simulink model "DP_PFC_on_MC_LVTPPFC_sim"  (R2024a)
settings: Solver=odeN  StartTime=0.0  StopTime=1  FixedStep=Ts  MaxStep=10e-6  RelTol=1e-3  AbsTol=1e-4  EnableMultiTasking=on
PreLoadFcn:
  | TotemPole_PFCData;
StopFcn:
  | out.getSimulationMetadata.TimingInfo
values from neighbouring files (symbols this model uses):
  PWM = PWMType.Implementation    [TotemPole_PFCData.m]
  Ts = 5e-9    (= 5e-09)    [TotemPole_PFCData.m]
  Tsc_fast = 1e-5    (= 1e-05)    [TotemPole_PFCData.m]
  Tsc_slow = 0.01    [TotemPole_PFCData.m]
  Vrms = 23.0    (= 23)    [TotemPole_PFCData.m]
undefined symbols (not defined in the file or in its folder): AC, ADCs, ClosedLoop, Const, Detailed, Implementation, Inversion, Microchip, Noise, PI, Rnom, Simulation, ZenerResistiveLoad
libraries: fl_lib x23, nesl_utility x15, ee_lib x11, simulink x8, slctrl_fre x1, eeTotalHarmonicDistorsion x1
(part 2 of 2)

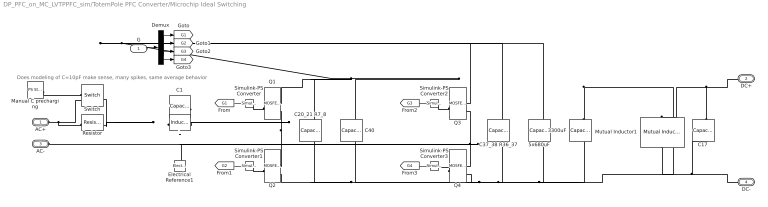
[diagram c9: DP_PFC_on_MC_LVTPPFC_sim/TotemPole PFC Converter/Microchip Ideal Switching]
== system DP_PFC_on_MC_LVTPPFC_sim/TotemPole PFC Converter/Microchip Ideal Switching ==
  note: Does modeling of C=10pF make sense, many spikes, same average behavior
  G : Inport
  3300uF : fl_lib/Electrical/Electrical Elements/Capacitor  c=3300 uF  r=65 mOhm  g=0 1/Ohm  i_specify=off  i_priority=None  i=0 A  i_nominal_specify=off  i_nominal_value=1  i_nominal_unit=A  v_specify=off  v_priority=High  v=0.1 V  v_nominal_specify=off  v_nominal_value=1  v_nominal_unit=V  vc_specify=off  vc_priority=High  vc=0 V  vc_nominal_specify=off  vc_nominal_value=1  vc_nominal_unit=V
  5x680uF : fl_lib/Electrical/Electrical Elements/Capacitor  c=680*5 uF  r=90/5 mOhm  g=0 1/Ohm  i_specify=off  i_priority=None  i=0 A  i_nominal_specify=off  i_nominal_value=1  i_nominal_unit=A  v_specify=off  v_priority=High  v=0.1 V  v_nominal_specify=off  v_nominal_value=1  v_nominal_unit=V  vc_specify=off  vc_priority=High  vc=0 V  vc_nominal_specify=off  vc_nominal_value=1  vc_nominal_unit=V
  C1 : fl_lib/Electrical/Electrical Elements/Capacitor  Commented=on  c=10 pF  r=0 Ohm  g=0 1/Ohm  i_specify=off  i_priority=None  i=0 A  i_nominal_specify=off  i_nominal_value=1  i_nominal_unit=A  v_specify=off  v_priority=High  v=0.1 V  v_nominal_specify=off  v_nominal_value=1  v_nominal_unit=V  vc_specify=off  vc_priority=High  vc=0 V  vc_nominal_specify=off  vc_nominal_value=1  vc_nominal_unit=V
  C17 : fl_lib/Electrical/Electrical Elements/Capacitor  c=2 uF  r=0 mOhm  g=0 1/Ohm  i_specify=off  i_priority=None  i=0 A  i_nominal_specify=off  i_nominal_value=1  i_nominal_unit=A  v_specify=off  v_priority=High  v=0.1 V  v_nominal_specify=off  v_nominal_value=1  v_nominal_unit=V  vc_specify=off  vc_priority=High  vc=0 V  vc_nominal_specify=off  vc_nominal_value=1  vc_nominal_unit=V
  C20_21 R7_8 : fl_lib/Electrical/Electrical Elements/Capacitor  c=44 nF  r=7.5 Ohm  g=0 1/Ohm  i_specify=off  i_priority=None  i=0 A  i_nominal_specify=off  i_nominal_value=1  i_nominal_unit=A  v_specify=off  v_priority=High  v=0.1 V  v_nominal_specify=off  v_nominal_value=1  v_nominal_unit=V  vc_specify=off  vc_priority=High  vc=0 V  vc_nominal_specify=off  vc_nominal_value=1  vc_nominal_unit=V
  C37_38 R36_37 : fl_lib/Electrical/Electrical Elements/Capacitor  c=44 nF  r=7.5 Ohm  g=0 1/Ohm  i_specify=off  i_priority=None  i=0 A  i_nominal_specify=off  i_nominal_value=1  i_nominal_unit=A  v_specify=off  v_priority=High  v=0.1 V  v_nominal_specify=off  v_nominal_value=1  v_nominal_unit=V  vc_specify=off  vc_priority=High  vc=0 V  vc_nominal_specify=off  vc_nominal_value=1  vc_nominal_unit=V
  C40 : fl_lib/Electrical/Electrical Elements/Capacitor  c=2 uF  r=0 mOhm  g=0 1/Ohm  i_specify=off  i_priority=None  i=0 A  i_nominal_specify=off  i_nominal_value=1  i_nominal_unit=A  v_specify=off  v_priority=High  v=0.1 V  v_nominal_specify=off  v_nominal_value=1  v_nominal_unit=V  vc_specify=off  vc_priority=High  vc=0 V  vc_nominal_specify=off  vc_nominal_value=1  vc_nominal_unit=V
  Demux : Demux
  Electrical Reference1 : fl_lib/Electrical/Electrical Elements/Electrical Reference
  L : fl_lib/Electrical/Electrical Elements/Inductor  l=266 uH  r=18 mOhm  g=0 1/Ohm  i_specify=off  i_priority=None  i=0 A  i_nominal_specify=off  i_nominal_value=1  i_nominal_unit=A  v_specify=off  v_priority=None  v=0 V  v_nominal_specify=off  v_nominal_value=1  v_nominal_unit=V  i_L_specify=off  i_L_priority=High  i_L=0 A  i_L_nominal_specify=off  i_L_nominal_value=1  i_L_nominal_unit=A
  Manual C precharging : fl_lib/Physical Signals/Sources/PS Step  step_time=0.10 ms  initial_value=1  final_value=0
  Mutual Inductor1 : ee_lib/Passive/Transformers/Mutual Inductor  L1=4.7 uH  L2=4.7 uH  k=0.9  L_tol=0  enable_L1_tol=ee.enum.toleranceApplication.none  L1_tol_distribution=ee.enum.toleranceDistribution.uniform  L1_nSigma=4  enable_L2_tol=ee.enum.toleranceApplication.none  L2_tol_distribution=ee.enum.toleranceDistribution.uniform  L2_nSigma=4  r=[4,4] mOhm  g=[1e-8,1e-8] 1/Ohm  enable_operating_limits=ee.enum.enable.no  operating_limit_action=ee.enum.passive.reportOpLim.warn  max_working_current=1 A  power_rating=1 W  enable_faults=ee.enum.enable.no  fault_action=simscape.enum.assert.action.none  fault_winding=ee.enum.passive.transformers.faultedWinding.primary  lambdaPercent=50  turnsShort=ee.enum.faults.faultTurnsShort.no  openCct=ee.enum.faults.faultTurnsOpenCkt.no  groundShort=ee.enum.faults.faultTurnsGroundShort.no  groundShortG=0 1/Ohm  tau_fault=1e-3 s  fault_trigger=ee.enum.faults.faultTrigger.temporal  t_fault=1 s  max_permissible_voltage=100 V  n_fail_on_voltage=1  max_permissible_current=1 A  t_fail_on_current=1 s  iL1_specify=off  iL1_priority=High  iL1=0 A  iL1_nominal_specify=off  iL1_nominal_value=1  iL1_nominal_unit=A  iL2_specify=off  iL2_priority=High  iL2=0 A  iL2_nominal_specify=off  iL2_nominal_value=1  iL2_nominal_unit=A  faulted_specify=off  faulted_priority=None  faulted=0
  Q1 : ee_lib/Semiconductors & Converters/MOSFET (Ideal, Switching)  port_option=ee.enum.controlport.ps  Rds=0.034 Ohm  Goff=1e-5 1/Ohm  Vth=0.5 V  diode_param=2  diode_Vf=3 V  diode_Ron=0.3 Ohm  diode_Goff=4e-5 1/Ohm  diode_C=50e-9 F  diode_iRM=-235 A  diode_iF=300 A  diode_idot=-50 A/us  diode_trr_param=1  diode_trr_factor=3  diode_trr=15 us  diode_Qrr=1500 s*uA  ids_specify=off  ids_priority=None  ids=0 A  ids_nominal_specify=off  ids_nominal_value=1  ids_nominal_unit=A  vds_specify=off  vds_priority=None  vds=0 V  vds_nominal_specify=off  vds_nominal_value=1  vds_nominal_unit=V  vgs_specify=off  vgs_priority=None  vgs=0 V  vgs_nominal_specify=off  vgs_nominal_value=1  vgs_nominal_unit=V  thermal_loss_option=ee.enum.converters.thermalLossOption.constantvalues  Von_data=[0, 1.8, 3.2, 6, 10, 16; 0, 2, 5.5, 9.5, 15, 25] V  Tj=[298.15, 448.15] K  Iout_data=[0, 20, 40, 60, 80, 100] A  Eon_data=[0, 55.04, 124.57, 235.53, 362.12; 0, 71.25, 161.25, 304.88, 468.75] * 1e-6 J  Eoff_data=[0, 18, 30, 56.1, 76.5; 0, 22.5, 37.5, 70.13, 95.63] * 1e-6 J  Eon_data_3D=[zeros(2, 5, 3)] J  Eoff_data_3D=[zeros(2, 5, 3)] J  Tj_loss=[298.15, 448.15] K  Iout_data_loss=[0, 10, 20, 30, 40] A  tabulateWithVds=false  Vds_loss=[0, 150, 300] V  Eon_scalar=22.86e-3 J  Eoff_scalar=17.14e-3 J  Voff=300 V  Iout_scalar=600 A  useCurrentFromPreviousCycle=false  useVoltageFromPreviousCycle=false  diodeModelType=ee.enum.converters.diodeModelType.pwl  diodeTableType=ee.enum.diode.tableType.IfMat  diode_ReverseIVType=ee.enum.diode.diodeReverseIV.constant  diode_IfMat=[.07, .12, .19, 1.75, 4.24, 7.32, 11.2; .16, .3, .72, 2.14, 4.02, 6.35, 9.12] A  diode_VfMat=[.9, 1.15, 1.25, 1.5, 1.75, 2.17, 2.6, 2.85; .58, .68, .75, 1.1, 1.38, 1.77, 2.27, 2.7] V  diode_TjVec=[25, 125] degC  diode_VfVec=[.5, .7, .9, 1.3, 1.7, 2.1, 2.5] V  diode_IfVec=[.1, .2, .5, 1, 2, 4, 7, 10] A  diode_IrMat=[1e-06, 2e-06, 5e-06, 1e-05, 2.5e-05, 5e-05, .0001; 2e-06, 5e-06, 1e-05, 4e-05, 8e-05, .0002, .0005] A  diode_VrMat=[10, 100, 200, 250, 300, 325, 350; 10, 70, 160, 220, 270, 300, 320] V  diode_VrVec=[10, 20, 40, 50, 70, 80, 100] V  diode_IrVec=[1e-06, 2e-06, 5e-06, 1e-05, 2e-05, 5e-05, .0001] A  diode_Vr=-600 V  diode_Ls=150 nH  diode_Erec=0.03 J  diode_rec_loss_model=ee.enum.diode.reverseRecoveryModel.fixed  diode_ErecVal=0 J  diode_scaleWithIandV=true  diode_ErecMat=zeros(2, 3) J  diode_TjrecVec=[298.15, 398.15] K  diode_IfrecVec=[.1, 1, 10] A  diode_IrecVal=10 A  diode_VrecVal=10 V  diode_tFilter=1 / 1000 / 100 s  thermal_network_parameterization=ee.enum.thermalNetworkTopology.external  Rth=[.03, .2] K/W  Rth_Cauer=[.03, .1, .2] K/W  Rth_Foster=[.03, .2] K/W  thermal_mass_parameterization=ee.enum.thermalNetwork.timeconstant  thermal_mass=[3, 25] J/K  thermal_mass_Cauer=[3, 10, 25] J/K  thermal_mass_Foster=[33, 50] J/K  thermal_time_constant=[.1, 5] s  thermal_time_constant_Cauer=[.1, 1, 5] s  thermal_time_constant_Foster=[1, 10] s  thermal_mass_initial_temperatures=[25, 25] degC  thermal_mass_initial_temperatures_Cauer=[25, 25, 25] degC  junction_thermal_mass=0.1 J/K  Tvec_initial_Foster=[25, 25, 25, 25] degC  no_thermal_network=0  junction_temperature_specify=off  junction_temperature_priority=None  junction_temperature=25 degC  junction_temperature_nominal_specify=off  junction_temperature_nominal_value=1  junction_temperature_nominal_unit=degC  Qj_specify=off  Qj_priority=None  Qj=0 W  Qj_nominal_specify=off  Qj_nominal_value=1  Qj_nominal_unit=W  accumulatedSwitchingLosses_specify=off  accumulatedSwitchingLosses_priority=None  accumulatedSwitchingLosses=0 J
  Q2 : ee_lib/Semiconductors & Converters/MOSFET (Ideal, Switching)  port_option=ee.enum.controlport.ps  Rds=0.034 Ohm  Goff=1e-5 1/Ohm  Vth=0.5 V  diode_param=2  diode_Vf=3 V  diode_Ron=0.3 Ohm  diode_Goff=4e-5 1/Ohm  diode_C=50e-9 F  diode_iRM=-235 A  diode_iF=300 A  diode_idot=-50 A/us  diode_trr_param=1  diode_trr_factor=3  diode_trr=15 us  diode_Qrr=1500 s*uA  ids_specify=off  ids_priority=None  ids=0 A  ids_nominal_specify=off  ids_nominal_value=1  ids_nominal_unit=A  vds_specify=off  vds_priority=None  vds=0 V  vds_nominal_specify=off  vds_nominal_value=1  vds_nominal_unit=V  vgs_specify=off  vgs_priority=None  vgs=0 V  vgs_nominal_specify=off  vgs_nominal_value=1  vgs_nominal_unit=V  thermal_loss_option=ee.enum.converters.thermalLossOption.constantvalues  Von_data=[0, 1.8, 3.2, 6, 10, 16; 0, 2, 5.5, 9.5, 15, 25] V  Tj=[298.15, 448.15] K  Iout_data=[0, 20, 40, 60, 80, 100] A  Eon_data=[0, 55.04, 124.57, 235.53, 362.12; 0, 71.25, 161.25, 304.88, 468.75] * 1e-6 J  Eoff_data=[0, 18, 30, 56.1, 76.5; 0, 22.5, 37.5, 70.13, 95.63] * 1e-6 J  Eon_data_3D=[zeros(2, 5, 3)] J  Eoff_data_3D=[zeros(2, 5, 3)] J  Tj_loss=[298.15, 448.15] K  Iout_data_loss=[0, 10, 20, 30, 40] A  tabulateWithVds=false  Vds_loss=[0, 150, 300] V  Eon_scalar=22.86e-3 J  Eoff_scalar=17.14e-3 J  Voff=300 V  Iout_scalar=600 A  useCurrentFromPreviousCycle=false  useVoltageFromPreviousCycle=false  diodeModelType=ee.enum.converters.diodeModelType.pwl  diodeTableType=ee.enum.diode.tableType.IfMat  diode_ReverseIVType=ee.enum.diode.diodeReverseIV.constant  diode_IfMat=[.07, .12, .19, 1.75, 4.24, 7.32, 11.2; .16, .3, .72, 2.14, 4.02, 6.35, 9.12] A  diode_VfMat=[.9, 1.15, 1.25, 1.5, 1.75, 2.17, 2.6, 2.85; .58, .68, .75, 1.1, 1.38, 1.77, 2.27, 2.7] V  diode_TjVec=[25, 125] degC  diode_VfVec=[.5, .7, .9, 1.3, 1.7, 2.1, 2.5] V  diode_IfVec=[.1, .2, .5, 1, 2, 4, 7, 10] A  diode_IrMat=[1e-06, 2e-06, 5e-06, 1e-05, 2.5e-05, 5e-05, .0001; 2e-06, 5e-06, 1e-05, 4e-05, 8e-05, .0002, .0005] A  diode_VrMat=[10, 100, 200, 250, 300, 325, 350; 10, 70, 160, 220, 270, 300, 320] V  diode_VrVec=[10, 20, 40, 50, 70, 80, 100] V  diode_IrVec=[1e-06, 2e-06, 5e-06, 1e-05, 2e-05, 5e-05, .0001] A  diode_Vr=-600 V  diode_Ls=150 nH  diode_Erec=0.03 J  diode_rec_loss_model=ee.enum.diode.reverseRecoveryModel.fixed  diode_ErecVal=0 J  diode_scaleWithIandV=true  diode_ErecMat=zeros(2, 3) J  diode_TjrecVec=[298.15, 398.15] K  diode_IfrecVec=[.1, 1, 10] A  diode_IrecVal=10 A  diode_VrecVal=10 V  diode_tFilter=1 / 1000 / 100 s  thermal_network_parameterization=ee.enum.thermalNetworkTopology.external  Rth=[.03, .2] K/W  Rth_Cauer=[.03, .1, .2] K/W  Rth_Foster=[.03, .2] K/W  thermal_mass_parameterization=ee.enum.thermalNetwork.timeconstant  thermal_mass=[3, 25] J/K  thermal_mass_Cauer=[3, 10, 25] J/K  thermal_mass_Foster=[33, 50] J/K  thermal_time_constant=[.1, 5] s  thermal_time_constant_Cauer=[.1, 1, 5] s  thermal_time_constant_Foster=[1, 10] s  thermal_mass_initial_temperatures=[25, 25] degC  thermal_mass_initial_temperatures_Cauer=[25, 25, 25] degC  junction_thermal_mass=0.1 J/K  Tvec_initial_Foster=[25, 25, 25, 25] degC  no_thermal_network=0  junction_temperature_specify=off  junction_temperature_priority=None  junction_temperature=25 degC  junction_temperature_nominal_specify=off  junction_temperature_nominal_value=1  junction_temperature_nominal_unit=degC  Qj_specify=off  Qj_priority=None  Qj=0 W  Qj_nominal_specify=off  Qj_nominal_value=1  Qj_nominal_unit=W  accumulatedSwitchingLosses_specify=off  accumulatedSwitchingLosses_priority=None  accumulatedSwitchingLosses=0 J
  Q3 : ee_lib/Semiconductors & Converters/MOSFET (Ideal, Switching)  port_option=ee.enum.controlport.ps  Rds=0.24 Ohm  Goff=1e-5 1/Ohm  Vth=0.5 V  diode_param=2  diode_Vf=3.6 V  diode_Ron=0.066 Ohm  diode_Goff=4e-5 1/Ohm  diode_C=50e-9 F  diode_iRM=-235 A  diode_iF=300 A  diode_idot=-50 A/us  diode_trr_param=1  diode_trr_factor=3  diode_trr=15 us  diode_Qrr=1500 s*uA  ids_specify=off  ids_priority=None  ids=0 A  ids_nominal_specify=off  ids_nominal_value=1  ids_nominal_unit=A  vds_specify=off  vds_priority=None  vds=0 V  vds_nominal_specify=off  vds_nominal_value=1  vds_nominal_unit=V  vgs_specify=off  vgs_priority=None  vgs=0 V  vgs_nominal_specify=off  vgs_nominal_value=1  vgs_nominal_unit=V  thermal_loss_option=ee.enum.converters.thermalLossOption.constantvalues  Von_data=[0, 1.8, 3.2, 6, 10, 16; 0, 2, 5.5, 9.5, 15, 25] V  Tj=[298.15, 448.15] K  Iout_data=[0, 20, 40, 60, 80, 100] A  Eon_data=[0, 55.04, 124.57, 235.53, 362.12; 0, 71.25, 161.25, 304.88, 468.75] * 1e-6 J  Eoff_data=[0, 18, 30, 56.1, 76.5; 0, 22.5, 37.5, 70.13, 95.63] * 1e-6 J  Eon_data_3D=[zeros(2, 5, 3)] J  Eoff_data_3D=[zeros(2, 5, 3)] J  Tj_loss=[298.15, 448.15] K  Iout_data_loss=[0, 10, 20, 30, 40] A  tabulateWithVds=false  Vds_loss=[0, 150, 300] V  Eon_scalar=22.86e-3 J  Eoff_scalar=17.14e-3 J  Voff=300 V  Iout_scalar=600 A  useCurrentFromPreviousCycle=false  useVoltageFromPreviousCycle=false  diodeModelType=ee.enum.converters.diodeModelType.pwl  diodeTableType=ee.enum.diode.tableType.IfMat  diode_ReverseIVType=ee.enum.diode.diodeReverseIV.constant  diode_IfMat=[.07, .12, .19, 1.75, 4.24, 7.32, 11.2; .16, .3, .72, 2.14, 4.02, 6.35, 9.12] A  diode_VfMat=[.9, 1.15, 1.25, 1.5, 1.75, 2.17, 2.6, 2.85; .58, .68, .75, 1.1, 1.38, 1.77, 2.27, 2.7] V  diode_TjVec=[25, 125] degC  diode_VfVec=[.5, .7, .9, 1.3, 1.7, 2.1, 2.5] V  diode_IfVec=[.1, .2, .5, 1, 2, 4, 7, 10] A  diode_IrMat=[1e-06, 2e-06, 5e-06, 1e-05, 2.5e-05, 5e-05, .0001; 2e-06, 5e-06, 1e-05, 4e-05, 8e-05, .0002, .0005] A  diode_VrMat=[10, 100, 200, 250, 300, 325, 350; 10, 70, 160, 220, 270, 300, 320] V  diode_VrVec=[10, 20, 40, 50, 70, 80, 100] V  diode_IrVec=[1e-06, 2e-06, 5e-06, 1e-05, 2e-05, 5e-05, .0001] A  diode_Vr=-600 V  diode_Ls=150 nH  diode_Erec=0.03 J  diode_rec_loss_model=ee.enum.diode.reverseRecoveryModel.fixed  diode_ErecVal=0 J  diode_scaleWithIandV=true  diode_ErecMat=zeros(2, 3) J  diode_TjrecVec=[298.15, 398.15] K  diode_IfrecVec=[.1, 1, 10] A  diode_IrecVal=10 A  diode_VrecVal=10 V  diode_tFilter=1 / 1000 / 100 s  thermal_network_parameterization=ee.enum.thermalNetworkTopology.external  Rth=[.03, .2] K/W  Rth_Cauer=[.03, .1, .2] K/W  Rth_Foster=[.03, .2] K/W  thermal_mass_parameterization=ee.enum.thermalNetwork.timeconstant  thermal_mass=[3, 25] J/K  thermal_mass_Cauer=[3, 10, 25] J/K  thermal_mass_Foster=[33, 50] J/K  thermal_time_constant=[.1, 5] s  thermal_time_constant_Cauer=[.1, 1, 5] s  thermal_time_constant_Foster=[1, 10] s  thermal_mass_initial_temperatures=[25, 25] degC  thermal_mass_initial_temperatures_Cauer=[25, 25, 25] degC  junction_thermal_mass=0.1 J/K  Tvec_initial_Foster=[25, 25, 25, 25] degC  no_thermal_network=0  junction_temperature_specify=off  junction_temperature_priority=None  junction_temperature=25 degC  junction_temperature_nominal_specify=off  junction_temperature_nominal_value=1  junction_temperature_nominal_unit=degC  Qj_specify=off  Qj_priority=None  Qj=0 W  Qj_nominal_specify=off  Qj_nominal_value=1  Qj_nominal_unit=W  accumulatedSwitchingLosses_specify=off  accumulatedSwitchingLosses_priority=None  accumulatedSwitchingLosses=0 J
  Q4 : ee_lib/Semiconductors & Converters/MOSFET (Ideal, Switching)  port_option=ee.enum.controlport.ps  Rds=0.24 Ohm  Goff=1e-5 1/Ohm  Vth=0.5 V  diode_param=2  diode_Vf=3.6 V  diode_Ron=0.066 Ohm  diode_Goff=4e-5 1/Ohm  diode_C=50e-9 F  diode_iRM=-235 A  diode_iF=300 A  diode_idot=-50 A/us  diode_trr_param=1  diode_trr_factor=3  diode_trr=15 us  diode_Qrr=1500 s*uA  ids_specify=off  ids_priority=None  ids=0 A  ids_nominal_specify=off  ids_nominal_value=1  ids_nominal_unit=A  vds_specify=off  vds_priority=None  vds=0 V  vds_nominal_specify=off  vds_nominal_value=1  vds_nominal_unit=V  vgs_specify=off  vgs_priority=None  vgs=0 V  vgs_nominal_specify=off  vgs_nominal_value=1  vgs_nominal_unit=V  thermal_loss_option=ee.enum.converters.thermalLossOption.constantvalues  Von_data=[0, 1.8, 3.2, 6, 10, 16; 0, 2, 5.5, 9.5, 15, 25] V  Tj=[298.15, 448.15] K  Iout_data=[0, 20, 40, 60, 80, 100] A  Eon_data=[0, 55.04, 124.57, 235.53, 362.12; 0, 71.25, 161.25, 304.88, 468.75] * 1e-6 J  Eoff_data=[0, 18, 30, 56.1, 76.5; 0, 22.5, 37.5, 70.13, 95.63] * 1e-6 J  Eon_data_3D=[zeros(2, 5, 3)] J  Eoff_data_3D=[zeros(2, 5, 3)] J  Tj_loss=[298.15, 448.15] K  Iout_data_loss=[0, 10, 20, 30, 40] A  tabulateWithVds=false  Vds_loss=[0, 150, 300] V  Eon_scalar=22.86e-3 J  Eoff_scalar=17.14e-3 J  Voff=300 V  Iout_scalar=600 A  useCurrentFromPreviousCycle=false  useVoltageFromPreviousCycle=false  diodeModelType=ee.enum.converters.diodeModelType.pwl  diodeTableType=ee.enum.diode.tableType.IfMat  diode_ReverseIVType=ee.enum.diode.diodeReverseIV.constant  diode_IfMat=[.07, .12, .19, 1.75, 4.24, 7.32, 11.2; .16, .3, .72, 2.14, 4.02, 6.35, 9.12] A  diode_VfMat=[.9, 1.15, 1.25, 1.5, 1.75, 2.17, 2.6, 2.85; .58, .68, .75, 1.1, 1.38, 1.77, 2.27, 2.7] V  diode_TjVec=[25, 125] degC  diode_VfVec=[.5, .7, .9, 1.3, 1.7, 2.1, 2.5] V  diode_IfVec=[.1, .2, .5, 1, 2, 4, 7, 10] A  diode_IrMat=[1e-06, 2e-06, 5e-06, 1e-05, 2.5e-05, 5e-05, .0001; 2e-06, 5e-06, 1e-05, 4e-05, 8e-05, .0002, .0005] A  diode_VrMat=[10, 100, 200, 250, 300, 325, 350; 10, 70, 160, 220, 270, 300, 320] V  diode_VrVec=[10, 20, 40, 50, 70, 80, 100] V  diode_IrVec=[1e-06, 2e-06, 5e-06, 1e-05, 2e-05, 5e-05, .0001] A  diode_Vr=-600 V  diode_Ls=150 nH  diode_Erec=0.03 J  diode_rec_loss_model=ee.enum.diode.reverseRecoveryModel.fixed  diode_ErecVal=0 J  diode_scaleWithIandV=true  diode_ErecMat=zeros(2, 3) J  diode_TjrecVec=[298.15, 398.15] K  diode_IfrecVec=[.1, 1, 10] A  diode_IrecVal=10 A  diode_VrecVal=10 V  diode_tFilter=1 / 1000 / 100 s  thermal_network_parameterization=ee.enum.thermalNetworkTopology.external  Rth=[.03, .2] K/W  Rth_Cauer=[.03, .1, .2] K/W  Rth_Foster=[.03, .2] K/W  thermal_mass_parameterization=ee.enum.thermalNetwork.timeconstant  thermal_mass=[3, 25] J/K  thermal_mass_Cauer=[3, 10, 25] J/K  thermal_mass_Foster=[33, 50] J/K  thermal_time_constant=[.1, 5] s  thermal_time_constant_Cauer=[.1, 1, 5] s  thermal_time_constant_Foster=[1, 10] s  thermal_mass_initial_temperatures=[25, 25] degC  thermal_mass_initial_temperatures_Cauer=[25, 25, 25] degC  junction_thermal_mass=0.1 J/K  Tvec_initial_Foster=[25, 25, 25, 25] degC  no_thermal_network=0  junction_temperature_specify=off  junction_temperature_priority=None  junction_temperature=25 degC  junction_temperature_nominal_specify=off  junction_temperature_nominal_value=1  junction_temperature_nominal_unit=degC  Qj_specify=off  Qj_priority=None  Qj=0 W  Qj_nominal_specify=off  Qj_nominal_value=1  Qj_nominal_unit=W  accumulatedSwitchingLosses_specify=off  accumulatedSwitchingLosses_priority=None  accumulatedSwitchingLosses=0 J
  Resistor : fl_lib/Electrical/Electrical Elements/Resistor  R=1 Ohm  i_specify=off  i_priority=None  i=0 A  i_nominal_specify=off  i_nominal_value=1  i_nominal_unit=A  v_specify=off  v_priority=None  v=0 V  v_nominal_specify=off  v_nominal_value=1  v_nominal_unit=V
  Simulink-PS Converter{,1..3} (4 alike) : nesl_utility/Simulink-PS Converter  PhysicalDomain=network_engine_domain  SubClassName=ps_input  LeftPortType=input  RightPortType=output  PseudoPeriodic=off  Frequencies=[]  NoiseDistribution=none  NoiseParameters=[]  Unit=1  AffineConversion=off  FilteringAndDerivatives=provide  SimscapeFilterOrder=1  InputFilterTimeConstant=0.001  UdotUserProvided=0
  Switch : fl_lib/Electrical/Electrical Elements/Switch  R_closed=0.0001 Ohm  G_open=1e-8 1/Ohm  Threshold=0.5  i_specify=off  i_priority=None  i=0 A  i_nominal_specify=off  i_nominal_value=1  i_nominal_unit=A  v_specify=off  v_priority=None  v=0 V  v_nominal_specify=off  v_nominal_value=1  v_nominal_unit=V
  AC+ : PMIOPort  Side=Left
  DC+ : PMIOPort  Port=2  Side=Right
  AC- : PMIOPort  Port=3  Side=Left
  DC- : PMIOPort  Port=4  Side=Right
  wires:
  G/1 -> Demux/1
  [G4] -> Simulink-PS Converter3/1
  [G2] -> Simulink-PS Converter1/1
  [G3] -> Simulink-PS Converter2/1
  [G1] -> Simulink-PS Converter/1
  Demux/3 -> [G3]
  Demux/2 -> [G2]
  Demux/1 -> [G1]
  Demux/4 -> [G4]
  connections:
  Q4/LConn1 -- Simulink-PS Converter3/RConn1
  Simulink-PS Converter2/RConn1 -- Q3/LConn1
  Simulink-PS Converter1/RConn1 -- Q2/LConn1
  Simulink-PS Converter/RConn1 -- Q1/LConn1
  Q2/RConn1 -- C1/LConn1 -- L/RConn1 -- Q1/RConn2
  Q3/RConn2 -- Electrical Reference1/LConn1 -- AC-/RConn1 -- Q4/RConn1
  C17/LConn1 -- DC+/RConn1 -- Mutual Inductor1/LConn1
  C20_21 R7_8/RConn1 -- Q2/RConn2 -- C40/RConn1 -- Q4/RConn2 -- C37_38 R36_37/RConn1 -- 5x680uF/RConn1 -- Mutual Inductor1/RConn2 -- 3300uF/RConn1
  3300uF/LConn1 -- Mutual Inductor1/LConn2 -- Q1/RConn1 -- C20_21 R7_8/LConn1 -- C40/LConn1 -- Q3/RConn1 -- C37_38 R36_37/LConn1 -- 5x680uF/LConn1
  Mutual Inductor1/RConn1 -- DC-/RConn1 -- C17/RConn1
  C1/RConn1 -- Switch/LConn1 -- Resistor/RConn1 -- L/LConn1
  AC+/RConn1 -- Switch/RConn2 -- Resistor/LConn1
  Manual C precharging/RConn1 -- Switch/RConn1

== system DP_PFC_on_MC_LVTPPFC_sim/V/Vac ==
  VinAC : fl_lib/Electrical/Electrical Sources/AC Voltage Source  amp=Vrms*sqrt(2) V  shift=0 deg  frequency=f_in Hz
  + : PMIOPort  Side=Left
  - : PMIOPort  Port=2  Side=Right
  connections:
  VinAC/RConn1 -- -/RConn1
  VinAC/LConn1 -- +/RConn1

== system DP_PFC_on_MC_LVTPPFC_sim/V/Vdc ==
  note: Used only for Bode Plot creation
  VinDC : ee_lib/Additional Components/SPICE Sources/DC Voltage Source  DC=30 V
  + : PMIOPort  Side=Left
  - : PMIOPort  Port=2  Side=Right
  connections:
  VinDC/LConn1 -- +/RConn1
  VinDC/RConn1 -- -/RConn1

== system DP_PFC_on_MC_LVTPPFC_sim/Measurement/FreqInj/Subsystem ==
  V~ : Inport
  Controlled Voltage Source : fl_lib/Electrical/Electrical Sources/Controlled Voltage Source
  Simulink-PS Converter : nesl_utility/Simulink-PS Converter  PhysicalDomain=network_engine_domain  SubClassName=ps_input  LeftPortType=input  RightPortType=output  PseudoPeriodic=off  Frequencies=[]  NoiseDistribution=none  NoiseParameters=[]  Unit=1  AffineConversion=off  FilteringAndDerivatives=provide  SimscapeFilterOrder=1  InputFilterTimeConstant=0.001  UdotUserProvided=0
  - : PMIOPort  Side=Left
  + : PMIOPort  Port=2  Side=Right
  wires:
  V~/1 -> Simulink-PS Converter/1
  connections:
  Simulink-PS Converter/RConn1 -- Controlled Voltage Source/RConn1
  Controlled Voltage Source/RConn2 -- -/RConn1
  Controlled Voltage Source/LConn1 -- +/RConn1

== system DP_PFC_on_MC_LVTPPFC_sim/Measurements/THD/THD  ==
  sig : Inport
  Total Harmonic Distortion : eeTotalHarmonicDistorsion/Total Harmonic Distortion  f=f_in  Ts=Ts
  THD : Outport
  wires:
  sig/1 -> Total Harmonic Distortion/1
  Total Harmonic Distortion/1 -> THD/1  "THD"

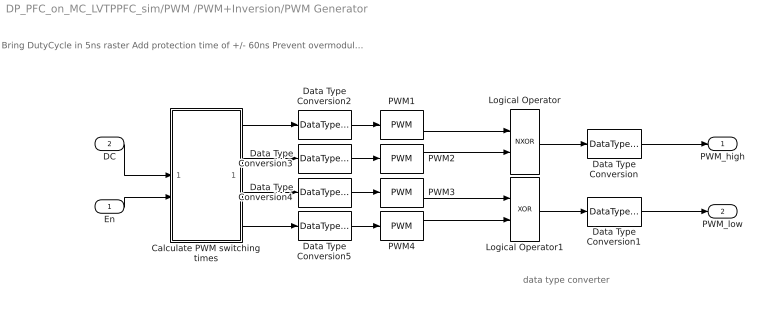
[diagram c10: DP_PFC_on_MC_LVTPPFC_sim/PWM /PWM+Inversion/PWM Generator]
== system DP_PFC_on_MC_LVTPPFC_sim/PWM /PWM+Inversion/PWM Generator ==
  note: data type converter
  note: Bring DutyCycle in 5ns raster Add protection time of +/- 60ns Prevent overmodulation
  En : Inport
  DC : Inport  Port=2
  Calculate PWM switching times : MATLAB Function  TreatAsAtomicUnit=on  mask{Tsc=10e-6, Ts=5e-9, DeadCycles=24}
      mask prompts: Tsc "PWM base time"; Ts "PWM Accuracy"; DeadCycles "Dead Cycles between High/Low rlated to accuracy (odd number)"
  Data Type Conversion{,1..5} (6 alike) : DataTypeConversion  OutDataTypeStr=double
  Logical Operator : Logic  Operator=NXOR  AllPortsSameDT=off  OutDataTypeStr=boolean
  Logical Operator1 : Logic  Operator=XOR  AllPortsSameDT=off  OutDataTypeStr=boolean
  PWM{1..4} (4 alike) : simulink/Discontinuities/PWM  DisableCoverage=on  Period=Tsc_fast  InitialDelay=0  DisallowZeroDutyCycle=off  RunAtFixedTimeIntervals=off  SampleTime=Ts
  PWM_high : Outport
  PWM_low : Outport  Port=2
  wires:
  PWM1/1 -> Logical Operator/1
  Calculate PWM switching times/1(dc_on_high) -> Data Type Conversion2/1
  PWM2/1 -> Logical Operator/2
  Logical Operator/1 -> Data Type Conversion/1
  DC/1 -> Calculate PWM switching times/1(DC)
  Calculate PWM switching times/2(dc_off_high) -> Data Type Conversion3/1
  Calculate PWM switching times/3(dc_on_low) -> Data Type Conversion4/1
  Calculate PWM switching times/4(dc_off_low) -> Data Type Conversion5/1
  PWM3/1 -> Logical Operator1/1
  PWM4/1 -> Logical Operator1/2
  Logical Operator1/1 -> Data Type Conversion1/1
  Data Type Conversion/1 -> PWM_high/1
  Data Type Conversion1/1 -> PWM_low/1
  En/1 -> Calculate PWM switching times/2(En)
  Data Type Conversion2/1 -> PWM1/1
  Data Type Conversion3/1 -> PWM2/1
  Data Type Conversion4/1 -> PWM3/1
  Data Type Conversion5/1 -> PWM4/1

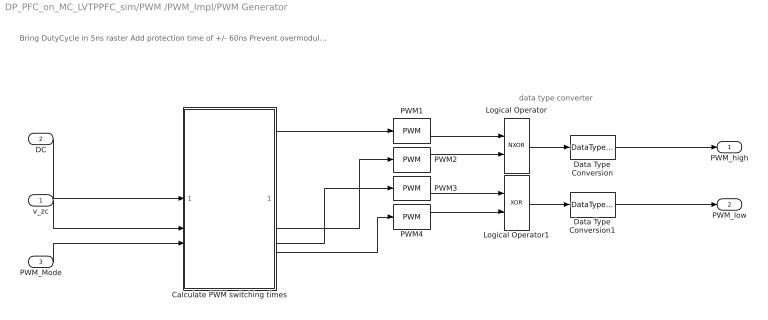
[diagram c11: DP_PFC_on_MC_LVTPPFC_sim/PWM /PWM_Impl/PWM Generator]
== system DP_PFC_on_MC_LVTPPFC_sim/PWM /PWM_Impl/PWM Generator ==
  note: Bring DutyCycle in 5ns raster Add protection time of +/- 60ns Prevent overmodulation
  note: data type converter
  v_zc : Inport
  DC : Inport  Port=2
  PWM_Mode : Inport  Port=3
  Calculate PWM switching times : MATLAB Function  TreatAsAtomicUnit=on  mask{Tsc=10e-6, Ts=5e-9, DeadCycles=24}
      mask prompts: Tsc "PWM base time"; Ts "PWM Accuracy"; DeadCycles "Dead Cycles between High/Low rlated to accuracy (odd number)"
  Data Type Conversion : DataTypeConversion  OutDataTypeStr=double
  Data Type Conversion1 : DataTypeConversion  OutDataTypeStr=double
  Logical Operator : Logic  Operator=NXOR  AllPortsSameDT=off  OutDataTypeStr=boolean
  Logical Operator1 : Logic  Operator=XOR  AllPortsSameDT=off  OutDataTypeStr=boolean
  PWM{1..4} (4 alike) : simulink/Discontinuities/PWM  DisableCoverage=on  Period=Tsc_fast  InitialDelay=0  DisallowZeroDutyCycle=off  RunAtFixedTimeIntervals=off  SampleTime=Ts
  PWM_high : Outport
  PWM_low : Outport  Port=2
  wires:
  Calculate PWM switching times/4(T_off_low) -> PWM4/1
  Calculate PWM switching times/3(T_on_low) -> PWM3/1
  Calculate PWM switching times/2(T_off_high) -> PWM2/1
  Calculate PWM switching times/1(T_on_high) -> PWM1/1
  Logical Operator1/1 -> Data Type Conversion1/1
  PWM4/1 -> Logical Operator1/2
  PWM3/1 -> Logical Operator1/1
  Logical Operator/1 -> Data Type Conversion/1
  PWM2/1 -> Logical Operator/2
  PWM1/1 -> Logical Operator/1
  Data Type Conversion/1 -> PWM_high/1
  Data Type Conversion1/1 -> PWM_low/1
  DC/1 -> Calculate PWM switching times/1(DC)
  v_zc/1 -> Calculate PWM switching times/2(v_zc)
  PWM_Mode/1 -> Calculate PWM switching times/3(PWM_Mode)

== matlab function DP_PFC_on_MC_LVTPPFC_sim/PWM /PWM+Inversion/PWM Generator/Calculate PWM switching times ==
function [dc_on_high,dc_off_high,dc_on_low,dc_off_low] = fcn(DC,En,Tsc_fast,Ts,DeadCycles)

if En
    % Output complementary PWM on high and low side with deadtime
    % Limit Duty Cycle to PWM accuracy
    Factor = Tsc_fast/Ts;
    DC = round(Factor*DC)/Factor;
   
    % Calculate switch on and off relative times for symmetrical PWM
    % related to low side switch
    dc_on = 0.5-DC/2;
    dc_off = 0.5+DC/2;
    
    dc_Dead = DeadCycles*Ts/Tsc_fast/2;
    
    dc_on_high = min(1,dc_off+dc_Dead);
    dc_off_high = max(0,dc_on-dc_Dead);
    
    dc_on_low = min(0.5,dc_on+dc_Dead);
    dc_off_low = max(0.5,dc_off-dc_Dead);
else
    % Set all gate drivers to 0 
    dc_on_low = single(0);
    dc_off_low = single(0);
    
    dc_on_high = single(0);
    dc_off_high = single(1);
end

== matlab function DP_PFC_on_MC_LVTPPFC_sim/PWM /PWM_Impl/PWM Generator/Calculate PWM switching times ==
function [T_on_high,T_off_high,T_on_low,T_off_low] = fcn(DC,v_zc,PWM_Mode,Tsc_fast,Ts,DeadCycles)

if v_zc || PWM_Mode == 12
      % Set all gate drivers to 0 
    T_on_low = 0.0;
    T_off_low = 0.0;
    
    T_on_high = 0.0;
    T_off_high = 1.0;

else
    % Output complementary PWM on high and low side with deadtime
    % Limit Duty Cycle to PWM accuracy
    Factor = Tsc_fast/Ts;
    DC = round(Factor*DC)/Factor;
   
    % Calculate switch on and off relative times for symmetrical PWM
    % related to low side switch
    T_on = 0.5-DC/2;
    T_off = 0.5+DC/2;
    
    T_Dead = DeadCycles*Ts/Tsc_fast/2;
    
    T_on_high = min(1,T_off+T_Dead);
    T_off_high = max(0,T_on-T_Dead);
    
    T_on_low = min(0.5,T_on+T_Dead);
    T_off_low = max(0.5,T_off-T_Dead);

    switch PWM_Mode
        case 0 % I > +I Threshold, no additional action
               % I < -I Threshold, no additional action
        

        case 8 % 0 <= I <= I Threshold : turn H off
            T_on_high = 0.0;
            T_off_high = 1.0;

        case 4 % -I Threshold <= I <= 0 : turn L off
            T_on_low = 0.0;
            T_off_low = 0.0;
    
        
        otherwise % no additional action
        
    end

end
